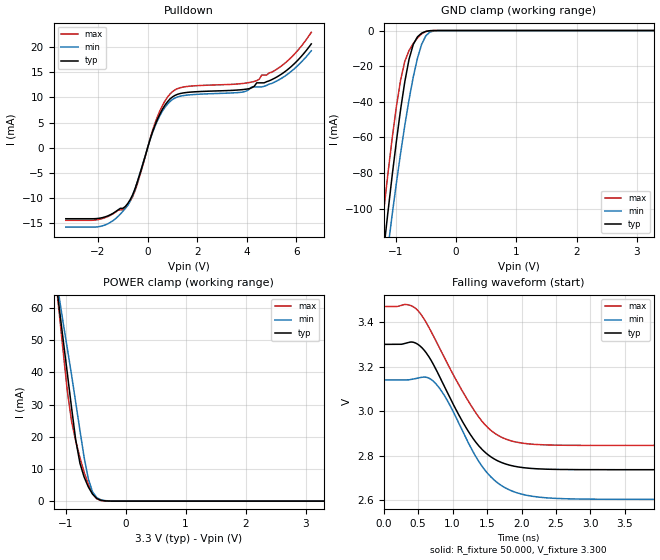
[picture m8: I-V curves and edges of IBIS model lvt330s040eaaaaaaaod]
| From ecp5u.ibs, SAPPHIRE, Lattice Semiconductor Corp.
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|   Model lvt330s040eaaaaaaaod
[Model] lvt330s040eaaaaaaaod
Model_type I/O_open_drain
Polarity   Non-Inverting
Enable   Active-Low
Vinl =  0.800V
Vinh =  2.000V
Vmeas =  1.650V
Cref =  0.0F
Rref =  1.000M
Vref =  3.3V
C_comp   5.000pF   4.000pF   5.500pF
[Temperature Range]   25.000   0.125k   -40.000
[Voltage Range]   3.300V   3.140V   3.470V
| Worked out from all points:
|   slope of the pulldown table from 0 to 0.495 V, typ, clamps not added: 73.9 ohm
|   GND clamp passes 1 mA (typ) near -0.54 V on its own axis
|   POWER clamp passes 1 mA (typ) near -0.49 V on its own axis
|   falling waveform, R_fixture 50.000, V_fixture 3.300: 20-80 % time 606ps typ, 585ps min, 676ps max; typ from 3.3 V to 2.74 V
[Pulldown]
|Voltage   I(typ)   I(min)   I(max)
-3.3V     -14.12mA   -15.79mA   -14.44mA
-1.8V     -13.87mA   -15.5mA    -14.05mA
-800mV    -11.08mA   -11.47mA   -11.33mA
-500mV    -8.065mA   -8.084mA   -8.464mA
300mV     4.505mA    4.281mA    4.905mA
600mV     7.672mA    7.282mA    8.406mA
1V        10.09mA    9.572mA    11.13mA
1.6V      10.99mA    10.46mA    12.17mA
4V        11.65mA    11.3mA     12.87mA
4.4V      12.89mA    12.07mA    13.33mA
5.5V      14.97mA    14.11mA    16.65mA
6.6V      20.62mA    19.27mA    22.93mA
[GND_clamp]
|Voltage   I(typ)   I(min)   I(max)
-3.3V     -912.7mA   -861.5mA   -922.5mA
-1.27V    -145.6mA   -163.6mA   -123.5mA
-1.2V     -123.4mA   -142.6mA   -101.4mA
-1.13V    -102mA     -122.4mA   -80.37mA
-1.06V    -81.56mA   -103.5mA   -60.64mA
-920mV    -44.4mA    -68.93mA   -27.87mA
-780mV    -16.18mA   -38.86mA   -11.24mA
-710mV    -7.839mA   -26.12mA   -7.318mA
-570mV    -1.464mA   -7.654mA   -1.852mA
-430mV    -105.8uA   -801.1uA   -99.73uA
-290mV    -1.56uA    -33.42uA   -868.4nA
3.28V     0A         0A         0A
[POWER_clamp]
|Voltage   I(typ)   I(min)   I(max)
-3.28V    471.5mA    421.2mA    516.6mA
-1.18V    71.72mA    72.75mA    72.14mA
-1.11V    60.88mA    63.98mA    59.38mA
-970mV    39.73mA    47.46mA    34.21mA
-900mV    29.12mA    39.28mA    24.89mA
-830mV    19.01mA    30.67mA    18.7mA
-760mV    11.8mA     22.01mA    13.51mA
-620mV    4.416mA    6.921mA    5.219mA
-550mV    2.174mA    2.865mA    2.414mA
-480mV    813uA      1.102mA    758.3uA
-200mV    3.62uA     22.61uA    424nA
3.3V      0A         0A         0A
[Ramp]
| variable   typ   min   max
dV/dt_r   0.338/1.202n   0.322/1.651n   0.375/0.445n
dV/dt_f   0.338/0.612n   0.322/0.595n   0.375/0.683n
R_load = 50.000
[Falling Waveform]
R_fixture= 50.000
V_fixture= 3.300
V_fixture_min= 3.140
V_fixture_max= 3.470
|time   V(typ)   V(min)   V(max)
0s        3.3V       3.14V      3.47V
429ps     3.31V      3.144V     3.469V
569ps     3.28V      3.153V     3.422V
716ps     3.213V     3.135V     3.341V
923ps     3.084V     3.047V     3.214V
1.353ns   2.853V     2.786V     2.984V
1.609ns   2.784V     2.688V     2.901V
1.933ns   2.75V      2.632V     2.86V
2.953ns   2.737V     2.604V     2.846V
10ns      2.736V     2.603V     2.846V
